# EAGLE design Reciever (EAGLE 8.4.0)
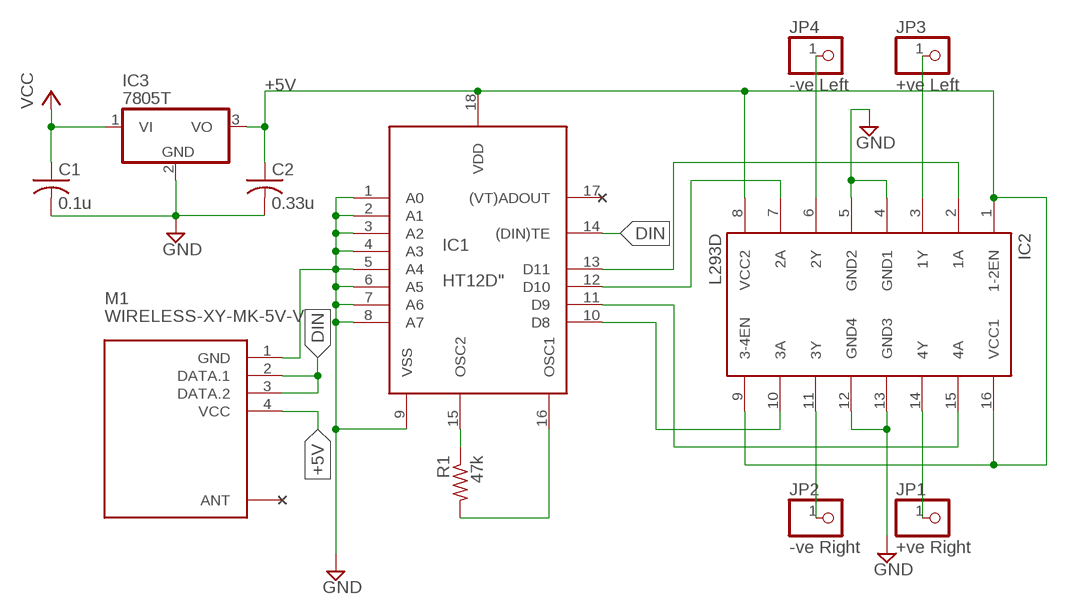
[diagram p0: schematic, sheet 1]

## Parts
C1  0.1u  C-USC0805  [C0805]
C2  0.33u  C-USC0805  [C0805]
IC1  HT12D"  [18-DIP-A]
IC2  L293D  [DIL16]
IC3  7805T  [TO220H]
JP1  +ve Right  PINHD-1X1  [1X01]
JP2  -ve Right  PINHD-1X1  [1X01]
JP3  +ve Left  PINHD-1X1  [1X01]
JP4  -ve Left  PINHD-1X1  [1X01]
M1  WIRELESS-XY-MK-5V-V  [WIRELESS-XY-MK-5V#V]
R1  47k  R-US_R0805  [R0805]

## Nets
+5V: C2.1 IC1.18(VDD) IC2.1(1-2EN) IC2.8(VCC2) IC2.9(3-4EN) IC2.16(VCC1) IC3.3(VO) M1.4(VCC)
DIN: IC1.14((DIN)TE) M1.2(DATA.1) M1.3(DATA.2)
GND: C1.2 C2.2 IC1.1(A0) IC1.2(A1) IC1.3(A2) IC1.4(A3) IC1.5(A4) IC1.6(A5) IC1.7(A6) IC1.8(A7) IC1.9(VSS) IC2.4(GND1) IC2.5(GND2) IC2.12(GND4) IC2.13(GND3) IC3.2(GND) M1.1(GND)
N$2: IC2.6(2Y) JP4.1
N$3: IC1.10(D8) IC2.10(3A)
N$4: IC1.15(OSC2) R1.1
N$5: IC1.16(OSC1) R1.2
N$6: IC1.11(D9) IC2.15(4A)
N$7: IC1.12(D10) IC2.7(2A)
N$8: IC1.13(D11) IC2.2(1A)
N$9: IC2.3(1Y) JP3.1
N$11: IC2.11(3Y) JP2.1
N$12: IC2.14(4Y) JP1.1
VCC: C1.1 IC3.1(VI)
Unconnected: IC1.17((VT)ADOUT) M1.ANT

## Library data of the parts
C1 C2 = adafruit:C-US: CAPACITOR, American symbol
IC1 = holtek:HT12D: decoder = receiver ic
IC2 = st-microelectronics:L293D: PUSH-PULL 4 CHANNEL DRIVER; MPN: L293D; OC_FARNELL: 9589619; OC_NEWARK: 56P8249
IC3 = adafruit:78*: Positive VOLTAGE REGULATOR Added bigger pads to the TO-92 package
JP1-JP4 = adafruit:PINHD-1X1: Pin header 1x1 for 0.1" spacing
M1 = diy-modules:WIRELESS-XY-MK-5V: RF Wireless XY-MK-5V Receiver Click here to find device on ebay.com Note: Sold together with transmitter.
R1 = adafruit:R-US_: RESISTOR, American symbol

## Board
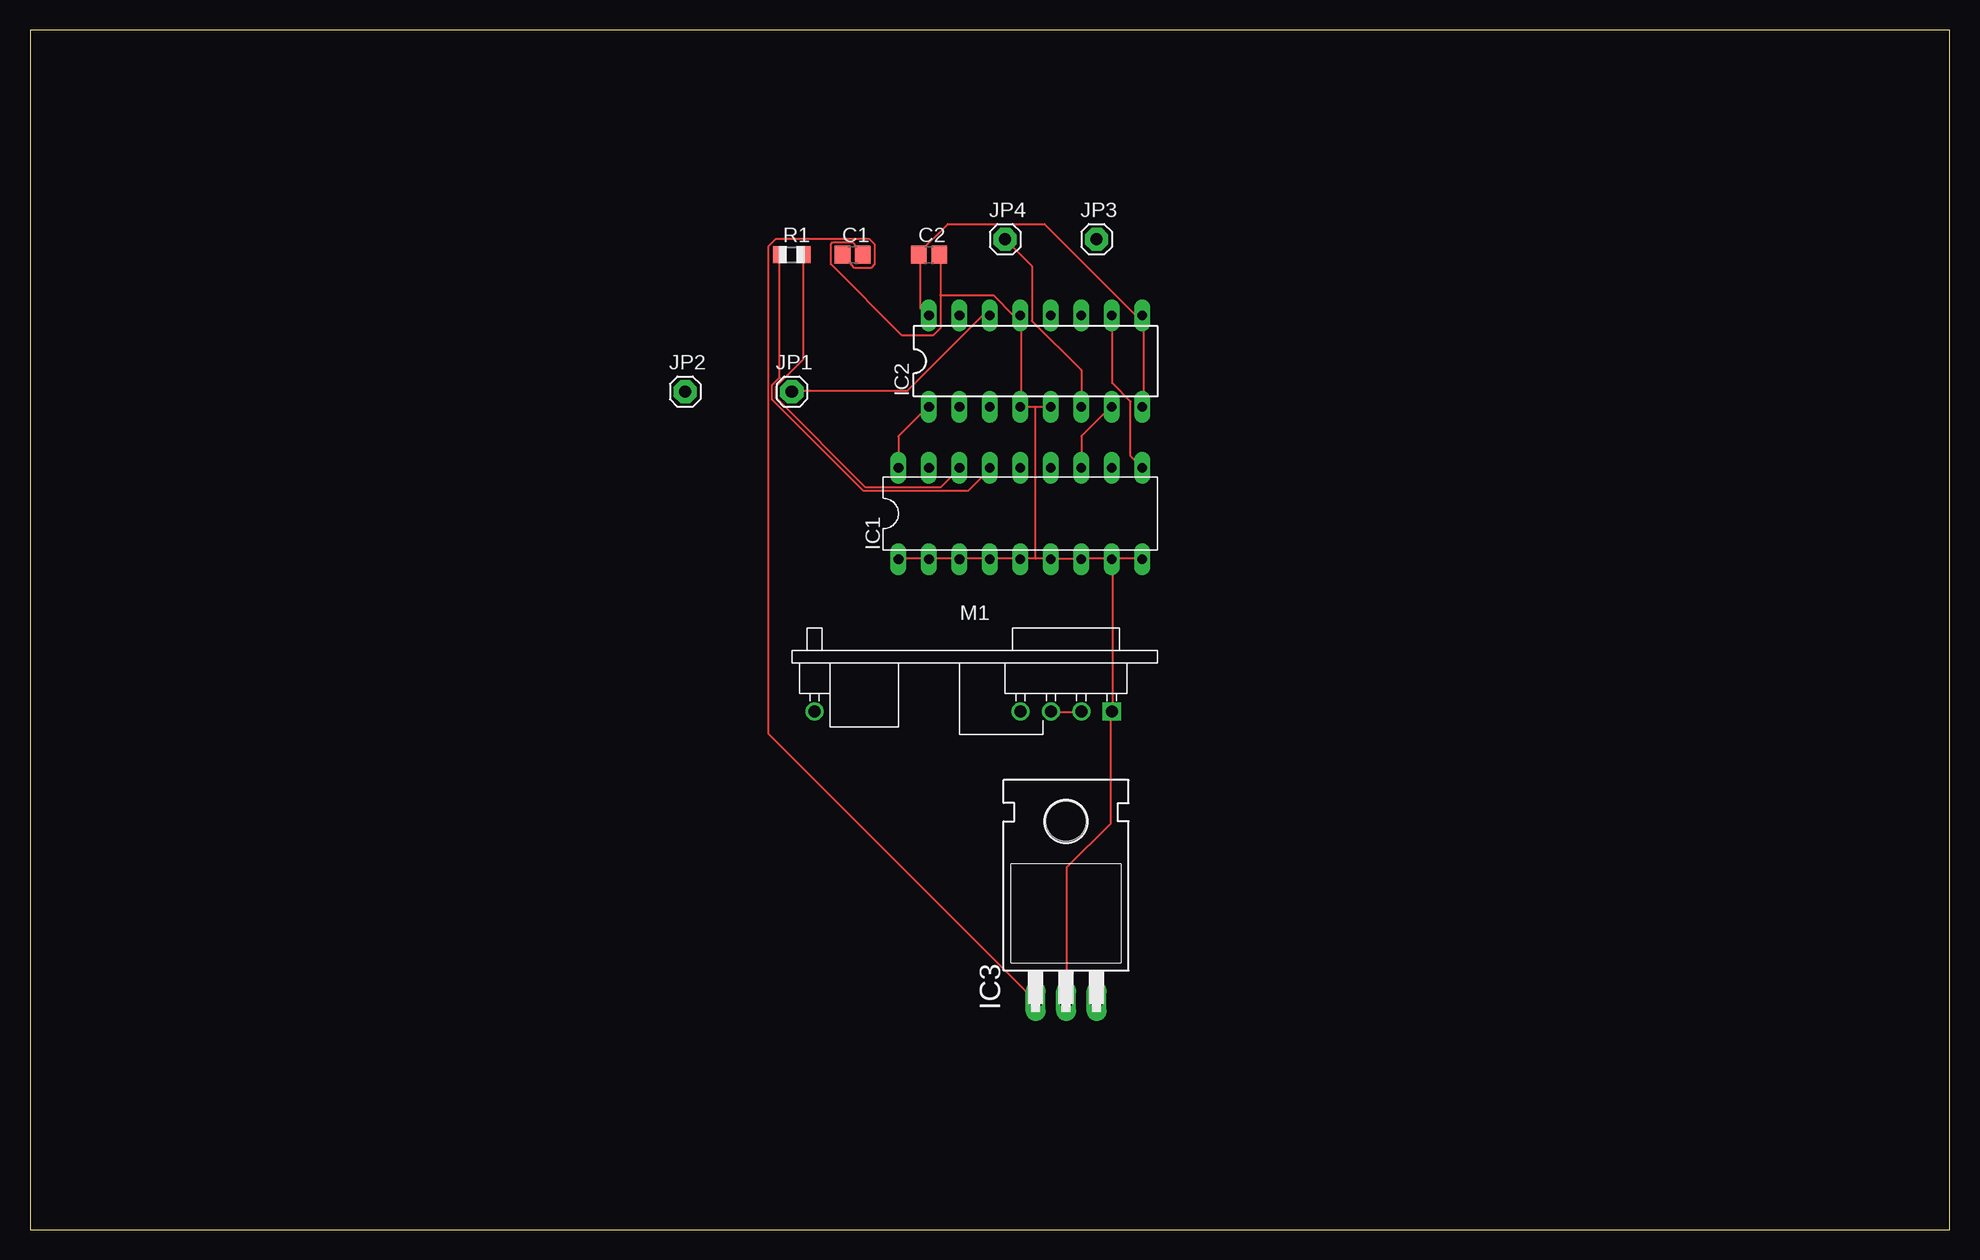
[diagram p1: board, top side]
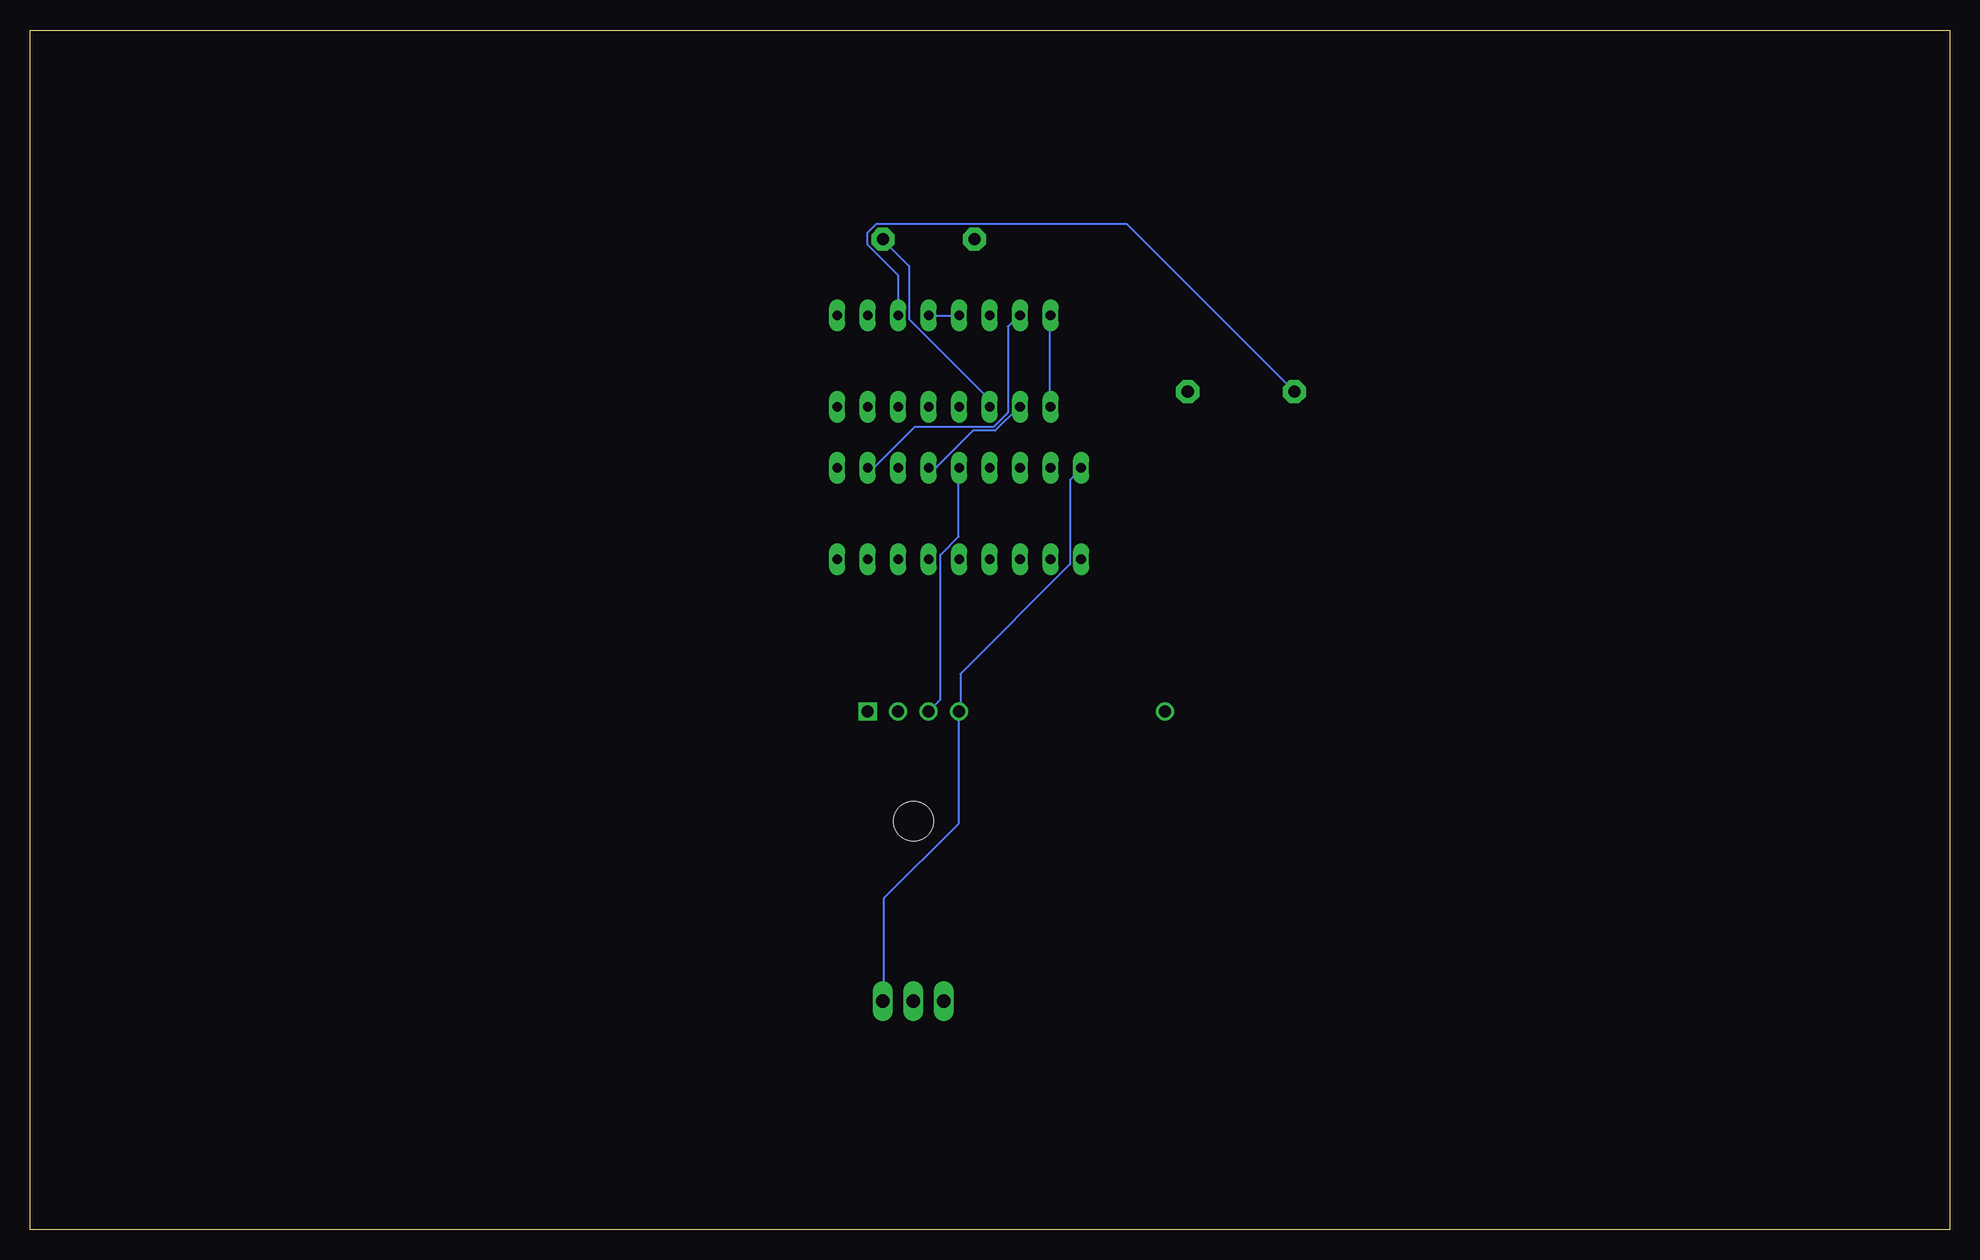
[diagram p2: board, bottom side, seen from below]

Size 160 x 100 mm. Coordinates in mm from the lower left corner, seen from the top.
Outline: 0,0 160,0 160,100 0,100 0,0
Copper layers (1*16): Top 0.035mm / dielectric 1.5mm / Bottom 0.035mm
Design rules "default": minimum track width 6mil, minimum drill 0.35mm, track to track 6mil, track to pad 6mil, pad to pad 6mil, via to via 6mil, smd to smd 6mil, copper to edge 40mil, drill to drill 6mil, minimum pad ring 10mil, minimum via ring 8mil, stop-mask expansion 4mil, vias tented up to drill 0mil, thermal gap 10mil

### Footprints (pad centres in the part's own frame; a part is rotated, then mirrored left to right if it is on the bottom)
C0805 = smd 1.3 x 1.5: 1 -0.85,0; 2 0.85,0
18-DIP-A = drill 0.813 long: 1 -10.16,-3.81; 2 -7.62,-3.81; 3 -5.08,-3.81; 4 -2.54,-3.81; 5 0,-3.81; 6 2.54,-3.81; 7 5.08,-3.81; 8 7.62,-3.81; 9 10.16,-3.81; 10 10.16,3.81; 11 7.62,3.81; 12 5.08,3.81; 13 2.54,3.81; 14 0,3.81; 15 -2.54,3.81; 16 -5.08,3.81; 17 -7.62,3.81; 18 -10.16,3.81
DIL16 = drill 0.813 long: 1 -8.89,-3.81; 2 -6.35,-3.81; 3 -3.81,-3.81; 4 -1.27,-3.81; 5 1.27,-3.81; 6 3.81,-3.81; 7 6.35,-3.81; 8 8.89,-3.81; 9 8.89,3.81; 10 6.35,3.81; 11 3.81,3.81; 12 1.27,3.81; 13 -1.27,3.81; 14 -3.81,3.81; 15 -6.35,3.81; 16 -8.89,3.81
TO220H = drill 1.118 long: 1 -2.54,-10.16; 2 0,-10.16; 3 2.54,-10.16 | hole 3.302: 0,4.826
1X01 = drill 1.016 pad 1.93 octagon: 1 0,0
WIRELESS-XY-MK-5V#V = drill 1 square: 1 11.43,0 | drill 1: 2 8.89,0; 3 6.35,0; 4 3.81,0; ANT -13.335,0
R0805 = smd 1.1 x 1.4: 1 -1,0; 2 1,0

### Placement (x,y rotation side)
C1  68.58,81.28 0 top
C2  74.93,81.28 0 top
IC1  82.55,59.69 0 top
IC2  83.82,72.39 0 top
IC3  86.36,29.21 0 top
JP1  63.5,69.85 0 top
JP2  54.61,69.85 0 top
JP3  88.9,82.55 0 top
JP4  81.28,82.55 0 top
M1  78.74,43.18 0 top
R1  63.5,81.28 0 top

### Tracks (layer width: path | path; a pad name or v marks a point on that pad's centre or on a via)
+5V
  Top 0.152: IC2.8 92.81,68.58 92.81,76.2 IC2.9 92.2,76.2 84.58,83.82 76.5,83.82 74.07,81.38 C2.1 74.22,81.23 74.22,76.81 74.83,76.2 IC2.16 | IC1.18 72.39,66.14 74.83,68.58 IC2.1
  Bottom 0.152: IC1.18 72.39,63.4 73.3,62.48 73.3,55.47 82.45,46.33 82.45,43.28 M1.4 82.6,43.13 82.6,33.83 88.85,27.58 88.85,19.05 IC3.3 | IC2.16 74.98,76.2 74.98,68.58 IC2.1
DIN
  Top 0.152: M1.2 87.63,43.13 85.19,43.13 M1.3
  Bottom 0.152: IC1.14 82.6,63.4 82.6,57.76 84.12,56.24 84.12,44.2 85.04,43.28 M1.3
GND
  Top 0.152: IC2.5 83.82,68.58 | 83.82,68.58 82.6,68.58 | 82.6,68.58 82.6,76.2 IC2.13 81.99,76.2 80.31,77.88 75.89,77.88 | 82.6,68.58 IC2.4 | 75.89,77.88 75.89,81.23 C2.2 | 75.89,77.88 75.89,75.13 75.29,74.52 72.69,74.52 66.75,80.47 66.75,82.14 66.9,82.3 68.58,82.3 68.73,82.14 68.73,81.99 69.34,81.38 C1.2 | IC1.1 72.39,55.93 74.83,55.93 IC1.2 74.98,55.93 77.42,55.93 IC1.3 77.57,55.93 80.01,55.93 | 83.82,55.93 85.04,55.93 IC1.6 85.19,55.93 87.63,55.93 | 83.82,55.93 82.6,55.93 IC1.5 82.45,55.93 80.01,55.93 | IC1.8 90.22,55.93 92.66,55.93 IC1.9 | IC1.8 90.22,55.78 90.22,43.28 M1.1 90.07,43.13 90.07,33.83 86.41,30.18 86.41,19.05 IC3.2 | 87.63,55.93 90.07,55.93 IC1.8 | 87.63,55.93 IC1.7 | 80.01,55.93 IC1.4 | 83.82,55.93 83.82,68.58
  Bottom 0.152: IC2.12 IC2.13
N$2
  Top 0.152: IC2.6 87.63,71.63 83.52,75.74 83.52,80.31 JP4.1
N$3
  Top 0.152: IC1.10 91.75,64.47 91.75,69.04 90.22,70.56 90.22,76.2 IC2.10
N$4
  Top 0.152: R1.1 62.48,81.23 62.48,71.02 61.87,70.41 61.87,69.19 69.49,61.57 78.18,61.57 80.01,63.4 IC1.15
N$5
  Top 0.152: R1.2 64.47,81.23 64.47,72.54 62.18,70.26 62.18,69.34 69.65,61.87 75.89,61.87 77.42,63.4 IC1.16
N$6
  Bottom 0.152: IC1.11 90.07,63.55 89.61,63.55 86.26,66.9 79.7,66.9 78.49,68.12 78.49,75.29 77.57,76.2 IC2.15
N$7
  Top 0.152: IC1.12 87.63,66.14 90.07,68.58 IC2.7
N$8
  Bottom 0.152: IC1.13 85.04,63.55 84.43,63.55 81.38,66.6 79.55,66.6 77.57,68.58 IC2.2
N$9
  Bottom 0.152: IC2.3 80.01,69.19 86.72,75.89 86.72,80.31 88.85,82.45 JP3.1
N$11
  Bottom 0.152: IC2.11 87.63,79.55 90.22,82.14 90.22,83.06 89.46,83.82 68.58,83.82 JP2.1
N$12
  Top 0.152: IC2.14 79.4,76.2 73.15,69.95 63.55,69.95 JP1.1
VCC
  Top 0.152: IC3.1 61.57,41.3 61.57,81.99 62.18,82.6 69.95,82.6 70.41,82.14 70.41,80.47 70.1,80.16 68.73,80.16 68.43,80.47 68.43,80.62 67.82,81.23 C1.1

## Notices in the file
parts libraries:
diy-modules: Released under the Creative Commons Attribution 4.0 International License: http://creativecommons.org/licenses/by/4.0
